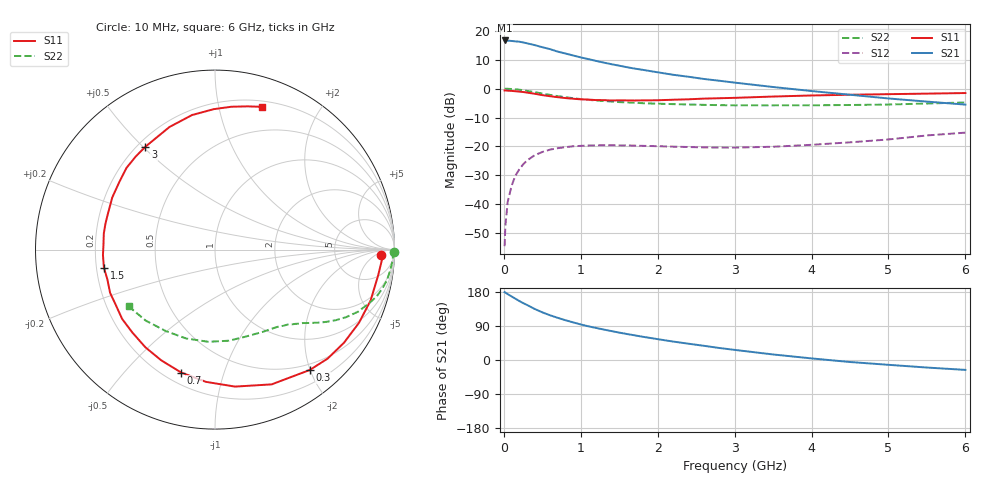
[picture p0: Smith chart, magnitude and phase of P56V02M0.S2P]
! SIEMENS Small Signal Semiconductors
! BFP183
! Si NPN RF Bipolar Junction Transistor in SOT143
! VCE = 6 V  IC = 2 mA
! Common Emitter S-Parameters:  March  1996
# GHz  S  MA  R  50
!  f  S11  S21  S12  S22
! GHz  MAG  ANG  MAG  ANG  MAG  ANG  MAG  ANG
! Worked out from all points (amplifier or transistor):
!   36 points, 10 MHz to 6 GHz, reference 50 ohm
!   highest |S21| = 16.6 dB at 10 MHz (marker M1)
!   |S21| within 3 dB of that: start of sweep to 600.9 MHz
!   unconditionally stable (mu >= 1): 2.142 GHz to 5.85 GHz
!   at 250 MHz: K = 0.12, MSG = 21.1 dB, |S12| = -26.2 dB
!   at 1.4 GHz: K = 0.66, MSG = 14.0 dB, |S12| = -19.6 dB
!   at 6 GHz: K = 0.97, MSG = 4.8 dB, |S12| = -15.2 dB
!   S11 on the Smith chart (normalised r, x): 10 MHz: 23, -9; 300 MHz: 0.40, -1.99; 700 MHz: 0.26, -0.73; 1.5 GHz: 0.23, -0.08; 3 GHz: 0.23, +0.51; 6 GHz: 0.25, +1.35
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0.01  0.9271 -1.7  6.778 178.9  0.0019 83.2  0.9991 -0.7
0.02  0.9315 -3.6  6.768 178.0  0.0043 88.4  0.9926 -1.3
0.05  0.9204 -8.9  6.734 173.9  0.011 87.3  0.9917 -3.3
0.1  0.9123 -18.0  6.648 167.8  0.0208 79.3  0.9832 -6.8
0.2  0.8865 -35.8  6.455 155.8  0.0402 70.1  0.9565 -13.2
0.25  0.8732 -44.1  6.266 150.2  0.049 65.3  0.9374 -16.2
0.3  0.8535 -51.8  6.063 145.4  0.0571 61.1  0.9128 -18.8
0.4  0.8145 -67.2  5.637 134.8  0.0705 53.3  0.8697 -23.4
0.5  0.7714 -81.7  5.186 125.8  0.0804 46.0  0.8213 -27.3
0.6  0.7386 -93.9  4.803 118.1  0.0883 40.4  0.7783 -30.4
0.7  0.7103 -105.4  4.347 111.3  0.0935 35.6  0.7408 -32.9
0.9  0.6685 -125.4  3.73 99.3  0.1009 27.9  0.6827 -36.7
1.1  0.6458 -143.2  3.228 88.8  0.1039 22.1  0.6381 -39.9
1.3  0.6322 -157.6  2.806 80.3  0.1052 17.7  0.6091 -42.8
1.5  0.627 -170.8  2.485 72.3  0.1044 14.8  0.5843 -45.4
1.8  0.626 171.7  2.113 61.5  0.1026 11.9  0.5599 -49.6
2.2  0.6419 153.1  1.733 48.7  0.0994 10.1  0.5391 -55.7
3  0.692 124.1  1.268 26.7  0.0956 13.5  0.5139 -70.7
3.5  0.7286 110.4  1.065 14.6  0.099 17.9  0.5136 -81.3
4.5  0.7826 90.5  0.783 -5.3  0.118 24.1  0.5207 -108.0
5.5  0.8184 77.2  0.596 -19.9  0.1552 24.6  0.5525 -134.2
6  0.8376 71.7  0.529 -26.1  0.1735 21.5  0.5757 -146.7
